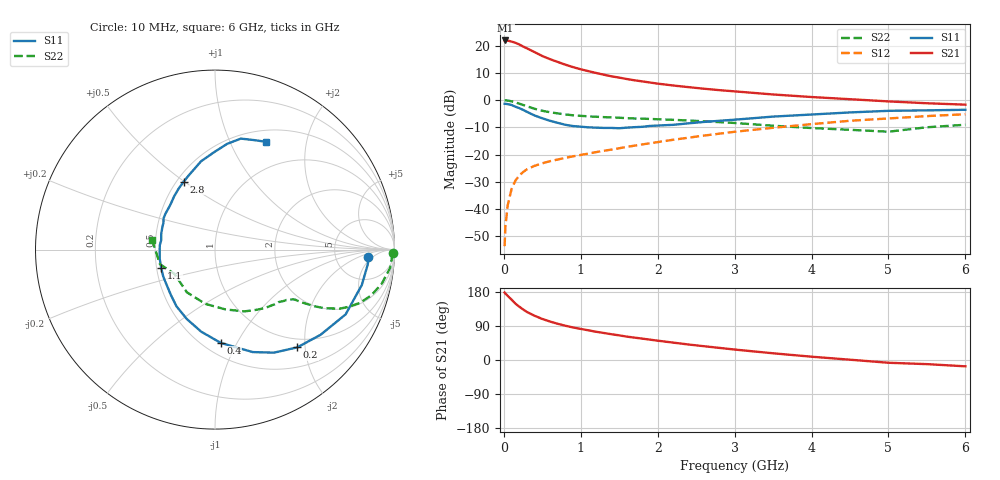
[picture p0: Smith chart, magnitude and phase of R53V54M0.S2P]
! SIEMENS Small Signal Semiconductors
! BFR183
! Si NPN RF Bipolar Junction Transistor in SOT23
! VCE = 3.5 V  IC = 4 mA
! Common Emitter S-Parameters:  May  1996
# GHz  S  MA  R  50
!  f  S11  S21  S12  S22
! GHz  MAG  ANG  MAG  ANG  MAG  ANG  MAG  ANG
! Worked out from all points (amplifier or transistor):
!   36 points, 10 MHz to 6 GHz, reference 50 ohm
!   highest |S21| = 21.9 dB at 20 MHz (marker M1)
!   |S21| within 3 dB of that: start of sweep to 307.9 MHz
!   unconditionally stable (mu >= 1): 1.142 GHz to 2.687 GHz
!   at 250 MHz: K = 0.36, MSG = 23.0 dB, |S12| = -26.4 dB
!   at 1.4 GHz: K = 1.06, MAG = 12.0 dB, |S12| = -18.1 dB
!   at 6 GHz: K = 0.89, MSG = 1.8 dB, |S12| = -5.2 dB
!   S11 on the Smith chart (normalised r, x): 10 MHz: 12, -4; 200 MHz: 0.84, -1.85; 400 MHz: 0.60, -0.86; 1.1 GHz: 0.53, -0.12; 2.8 GHz: 0.54, +0.50; 6 GHz: 0.64, +1.37
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0.01  0.8546 -2.8  12.2 178.0  0.0021 91.7  0.9921 -1.2
0.02  0.8555 -5.4  12.37 175.5  0.0048 85.1  0.9872 -2.4
0.05  0.8413 -13.6  12.32 169.2  0.0118 83.3  0.9808 -6.0
0.1  0.8123 -26.4  11.79 159.4  0.0233 77.3  0.9485 -11.5
0.15  0.7558 -38.9  11.23 148.9  0.0333 70.4  0.9075 -16.3
0.2  0.712 -49.9  10.45 140.8  0.0414 65.5  0.8599 -20.2
0.25  0.6616 -60.2  9.585 133.5  0.0479 61.8  0.8129 -23.0
0.3  0.6084 -69.8  8.871 126.8  0.0538 59.0  0.7696 -25.3
0.4  0.5212 -86.4  7.564 116.7  0.0624 55.2  0.6916 -28.2
0.5  0.4635 -99.6  6.415 108.3  0.0694 53.5  0.6362 -29.7
0.6  0.4174 -112.1  5.615 101.5  0.0758 52.5  0.5986 -30.5
0.7  0.3822 -124.1  4.998 95.6  0.0813 52.5  0.5698 -31.2
0.9  0.3342 -143.4  4.017 85.9  0.0932 53.7  0.5256 -32.0
1.1  0.3165 -161.6  3.384 78.3  0.1045 54.7  0.5035 -33.6
1.3  0.3086 -177.4  2.914 71.3  0.1176 55.4  0.4866 -35.2
1.6  0.3124 163.5  2.428 61.7  0.1387 56.8  0.4659 -38.5
2.2  0.3514 135.4  1.85 45.9  0.1871 56.5  0.4344 -47.4
2.8  0.4168 114.6  1.52 32.0  0.2419 53.2  0.3941 -59.6
3.5  0.4979 99.0  1.266 17.7  0.3104 46.5  0.3385 -80.0
4.5  0.5934 83.4  1.037 0.8  0.4173 34.9  0.2849 -123.4
5.5  0.6479 70.3  0.874 -10.9  0.5086 22.0  0.3173 -165.2
6  0.6637 64.9  0.824 -16.7  0.5502 13.6  0.3529 171.7
